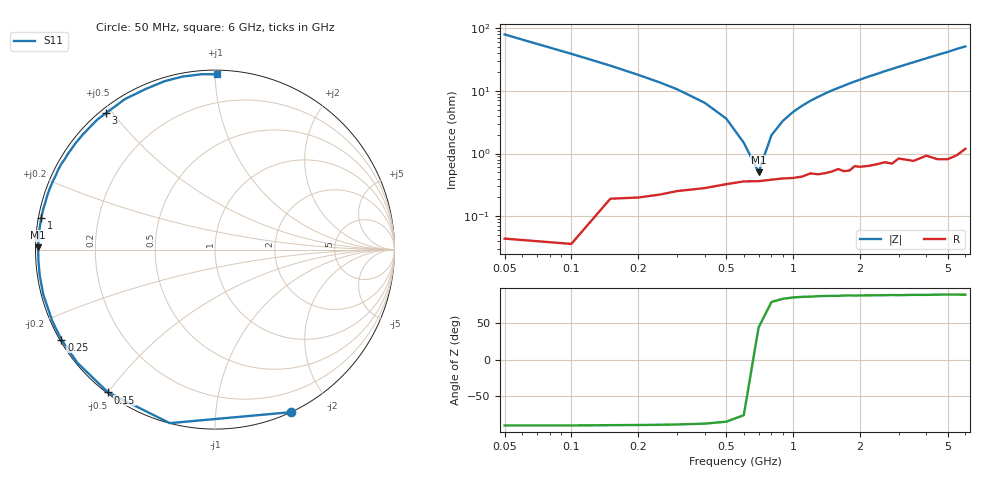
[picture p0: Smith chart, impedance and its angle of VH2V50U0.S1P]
! Infineon Technologies  Discrete & RF Semiconductors
! BB 814
! Si Tuning Diode in SOT23
! VR = 2.5 V
! S-Parameters:  July  1999
# GHz  S  MA  R  50
!  f  S11
! GHz  MAG  ANG
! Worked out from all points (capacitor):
!   34 points, 50 MHz to 6 GHz, reference 50 ohm
!   read as one part to ground: C = 40.3 pF near 50 MHz
!   lowest |Z| = 503 mohm at 700 MHz (marker M1)
!   series resonance near 680.5 MHz, so ESL is about 1.4 nH
!   S11 on the Smith chart (normalised r, x): 50 MHz: 0.00, -1.57; 150 MHz: 0.00, -0.50; 250 MHz: 0.00, -0.27; 1 GHz: 0.01, +0.09; 3 GHz: 0.02, +0.48; 6 GHz: 0.02, +1.01
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0.05  0.9995 -65.0
0.1  0.9991 -104.6
0.15  0.9939 -126.8
0.2  0.993 -140.6
0.25  0.9918 -149.6
0.3  0.9904 -156.2
0.4  0.989 -165.4
0.5  0.9872 -171.8
0.6  0.9857 -176.7
0.7  0.9856 179.2
0.8  0.9848 175.6
1  0.9839 169.6
1.3  0.9819 161.9
1.5  0.9803 157.2
1.6  0.9787 155.1
1.7  0.9804 153.0
1.9  0.9769 148.7
2.2  0.9774 142.8
2.4  0.9765 139.3
2.6  0.9754 135.5
2.8  0.9772 132.2
3  0.9733 128.7
3.5  0.9772 120.9
4  0.9745 113.5
4.5  0.9794 106.7
5  0.9809 100.7
5.5  0.9799 94.3
6  0.9768 89.2
